(* Logix 5000 AddOnInstructionDefinition export Process_TU3VFDControl_Instance102_103; software revision 24.02 *)

TYPE FI_Data_IN :
STRUCT
   ConnectionFaulted : BOOL;
   RunMode : BOOL;
   Data : INT[6];   // Actual Values
END_STRUCT
END_TYPE

TYPE FI_Data_OUT :
STRUCT
   Data : INT[6];   // Control Data
END_STRUCT
END_TYPE

ADD_ON_INSTRUCTION Process_TU3VFDControl_Instance102_103   (* revision 1.1, vendor NORD Drivesystems, ExecutePrescan *)
// Control block for Nord VFD TU3 Instances 102/103
// Allows for control of up to eight (8) SK 5xxE VFDs.
// Revision note:
// Rev 1.1
// Better Ready Start Condition Logic
// Added Inhibited Output
// Added Fault Active Output
// Rev 1.0
VAR_IN_OUT
   FI_Status : _0342:TU3_EIP_DE5BFA94:I:0; {required}   // Input Data Map of VFD
   FI_Control : _0342:TU3_EIP_E8E6FFA2:O:0; {required}   // Output Data Map of VFD
END_VAR
VAR_INPUT
   Max_VFD_Number : SINT := 8;   // Maximum Number of VFDs on this specific node (1-8 for Instance 102/103)
   VFD_Number : SINT := 1; {visible}   // Number of VFD to control (1...Max_VFD_Number) for Instance 102/103)
   EnableFwd : BOOL; {visible}   // HIGH = Enable CW
   EnableRev : BOOL; {visible}   // HIGH = Enable CCW
   DisableVoltage : BOOL := 1; {visible}   // LOW = Output Voltage Disabled
   QuickStop : BOOL := 1; {visible}   // LOW = Emergency Stop Active
   FaultAckn : BOOL; {visible}   // Error / Fault Acknowledgement on Rising Edge
   ParameterSet : SINT; {visible}   // Parameter Set 1-4, If less than 1 or higher than 4, Set 1 as active
   Activate32BitSetpoint : BOOL; {visible}   // HIGH = Activate 32Bit Setpoint combining Setpoint 2 and 3
   ControlWordBit8_P480_11 : BOOL; {visible}   // Control Word Bit 8 Function set in P480[11]
   ControlWordBit9_P480_12 : BOOL; {visible}   // Control Word Bit 9 Function set in P480[12]
END_VAR
VAR_OUTPUT
   ControlWord : ALIAS FOR Control_Word; {access Read Only, visible}   // Control Word Read Only Version
END_VAR
VAR_INPUT
   Setpoint1 : INT; {visible}   // Setpoint 1 Function set in P546
   Setpoint2 : INT; {visible}   // Setpoint 2 Function set in P547, deactivated if "PositioningActiveBit" is set
   Setpoint3 : INT; {visible}   // Setpoint 3 Function set in P548, deactivated if "PositioningActiveBitt" is set
   Setpoint4 : INT;   // Setpoint 4 only available in SK 54xE
   Setpoint5 : INT;   // Setpoint 5 only available in SK 54xE
   Setpoint2_3_32 : DINT; {visible}   // 32 Bit Setpoint 2 & 3 combined for positioning
END_VAR
VAR_OUTPUT
   StatusWord : INT; {access Read Only, visible}   // Status Word
        .0   // Ready to Start
        .1   // Ready for Operation
        .2   // Operation Enabled
        .3   // Fault
        .4   // Voltage Enabled
        .5   // No Emergency Stop
        .6   // Starting Disabled
        .7   // Warning Active
        .8   // Setpoint Reached
        .9   // Bus Controller Active
        .10   // Function P481[9]
        .11   // Rotation Right Active
        .12   // Rotation Left Active
        .13   // Function P481[10]
        .14   // Parameter Set Bit 0
        .15   // Parameter Set Bit 1
   ActiveParameterSet : SINT; {access None, visible}   // Displays Active Parameter set
   CommunicationOK : BOOL; {access Read Only, visible}   // HIGH = Communication is OK
   ReadyToStart : BOOL; {access None, visible}   // HIGH = Drive Ready to Start
   VFD_Enabled : BOOL; {access None, visible}   // HIGH = VFD is Enabled
   Inhibited : BOOL; {access Read Only, visible}   // VFD is Inhibited
   Warning : BOOL; {access None, visible}   // HIGH = Drive has a warning
   Faulted : BOOL; {access None, visible}   // HIGH = Drive Faulted
   FaultActive : BOOL; {access Read Only, visible}   // Fault Conditions are Currently Active
   StatusWordBit10_P481_9 : BOOL; {access None, visible}   // Status Word Bit 10 Function set in P481[9]
   StatusWordBit13_P481_10 : BOOL; {access None, visible}   // Status Word Bit 13 Function set in P481[10]
   ActualValue1 : INT; {access None, visible}   // Actual Value 1 Function set in P543
   ActualValue2 : INT; {access None, visible}   // Actual Value 2 Function set in P544
   ActualValue3 : INT; {access None, visible}   // Actual Value 3 Function set in P545
   ActualValue4 : INT; {access None}   // Actual Value 4 only available in SK 54xE
   ActualValue5 : INT; {access None}   // Actual Value 5 only available in SK 54xE
   ActualValue2_3_32 : DINT; {access None, visible}   // 32 Bit Actual Value 2 & 3 Combined for Positioning
END_VAR
VAR
   Index : INT; {access None}   // Index of process data based on VFD_Number
   Control_Word : INT; {access Read Only}   // Control Word
        .0   // Enable Operation
        .1   // Disable Voltage (Low level disables voltage and stops VFD)
        .2   // Emergency Stop (Low level activates ESTOP and stops VFD)
        .3   // Ready for Operation
        .4   // Enable Pulses
        .5   // Enable Ramp
        .6   // Enable Setpoint
        .7   // Error Acknowledge
        .8   // Function P480[11]
        .9   // Function P480[12]
        .10   // Control Data Valid
        .11   // Rotation Direction Right
        .12   // Rotation Direction Left
        .13   // Reserved
        .14   // Parameter Set Bit 0
        .15   // Parameter Set Bit 1
   Control : FI_Data_OUT; {access None}
   Status : FI_Data_IN; {access None}
   LowWordOf32BitSetpoint : DINT; {access None}
   Temporary_Variable_32BitSepoint : DINT; {access None}
   HighWordOf32BitSetpoint : DINT; {access None}
   FI_Status_Size : INT; {access None}   // Size of Input Process Data
   FI_Control_Size : INT; {access None}   // Size of Output Process Data
END_VAR

ROUTINE Logic   (* ladder *)
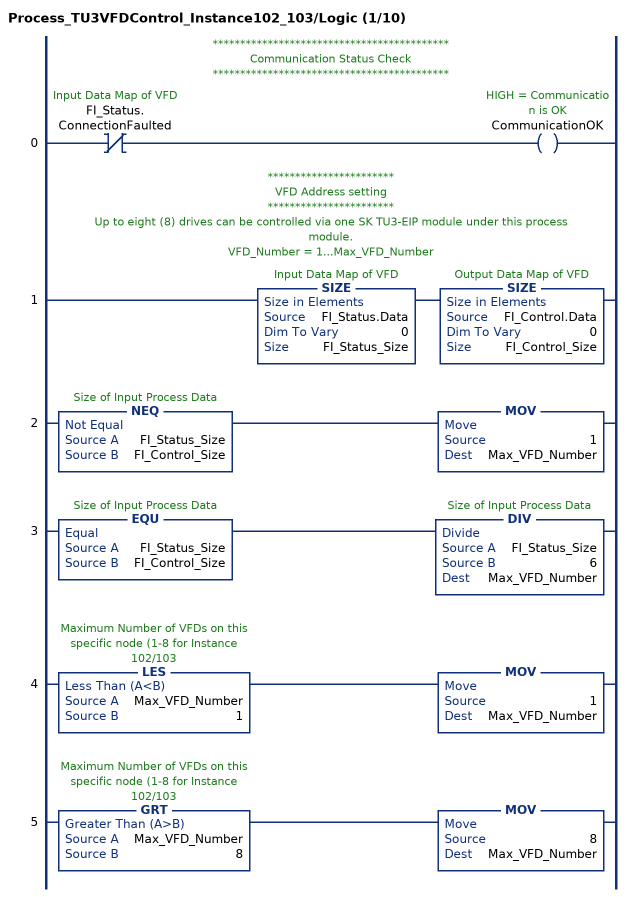
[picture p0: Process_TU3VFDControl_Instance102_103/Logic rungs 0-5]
   // *******************************************
   // Communication Status Check
   // *******************************************
   0: XIO(FI_Status.ConnectionFaulted)OTE(CommunicationOK);
   // ***********************
   // VFD Address setting
   // ***********************
   // Up to eight (8) drives can be controlled via one SK TU3-EIP module under this process module.
   // VFD_Number = 1...Max_VFD_Number
   1: SIZE(FI_Status.Data,0,FI_Status_Size)SIZE(FI_Control.Data,0,FI_Control_Size);
   2: NEQ(FI_Status_Size,FI_Control_Size)MOV(1,Max_VFD_Number);
   3: EQU(FI_Status_Size,FI_Control_Size)DIV(FI_Status_Size,6,Max_VFD_Number);
   4: LES(Max_VFD_Number,1)MOV(1,Max_VFD_Number);
   5: GRT(Max_VFD_Number,8)MOV(8,Max_VFD_Number);
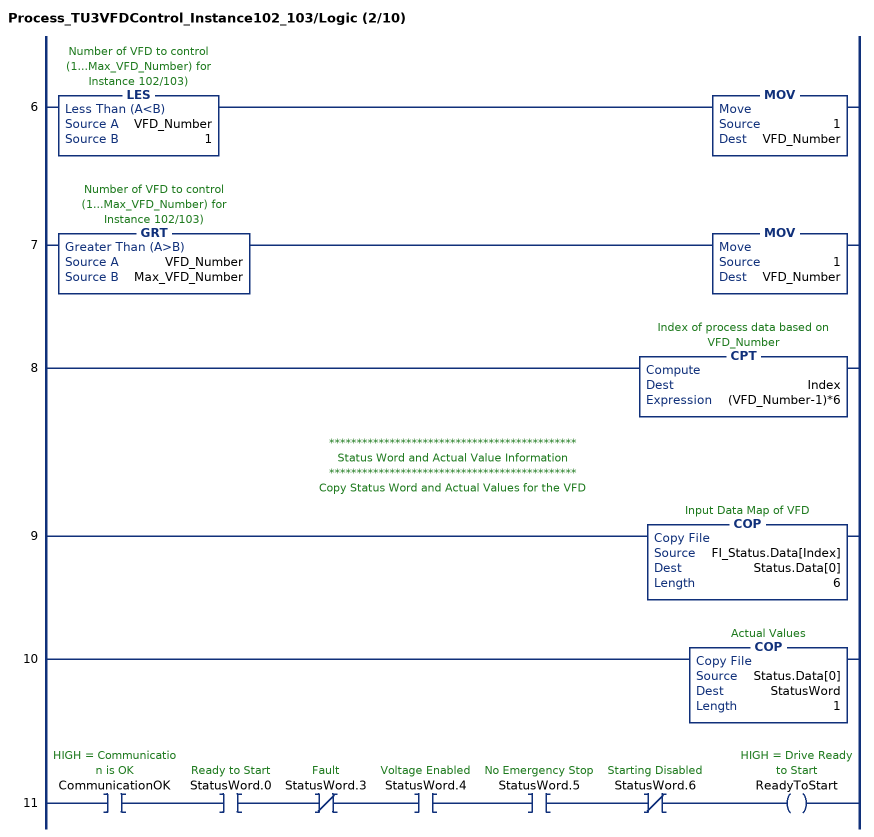
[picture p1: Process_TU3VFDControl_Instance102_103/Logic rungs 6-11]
   6: LES(VFD_Number,1)MOV(1,VFD_Number);
   7: GRT(VFD_Number,Max_VFD_Number)MOV(1,VFD_Number);
   8: CPT(Index,(VFD_Number-1)*6);
   // *********************************************
   // Status Word and Actual Value Information
   // *********************************************
   // Copy Status Word and Actual Values for the VFD
   9: COP(FI_Status.Data[Index],Status.Data[0],6);
   10: COP(Status.Data[0],StatusWord,1);
   11: XIC(CommunicationOK)XIC(StatusWord.0)XIO(StatusWord.3)XIC(StatusWord.4)XIC(StatusWord.5)XIO(StatusWord.6)OTE(ReadyToStart);
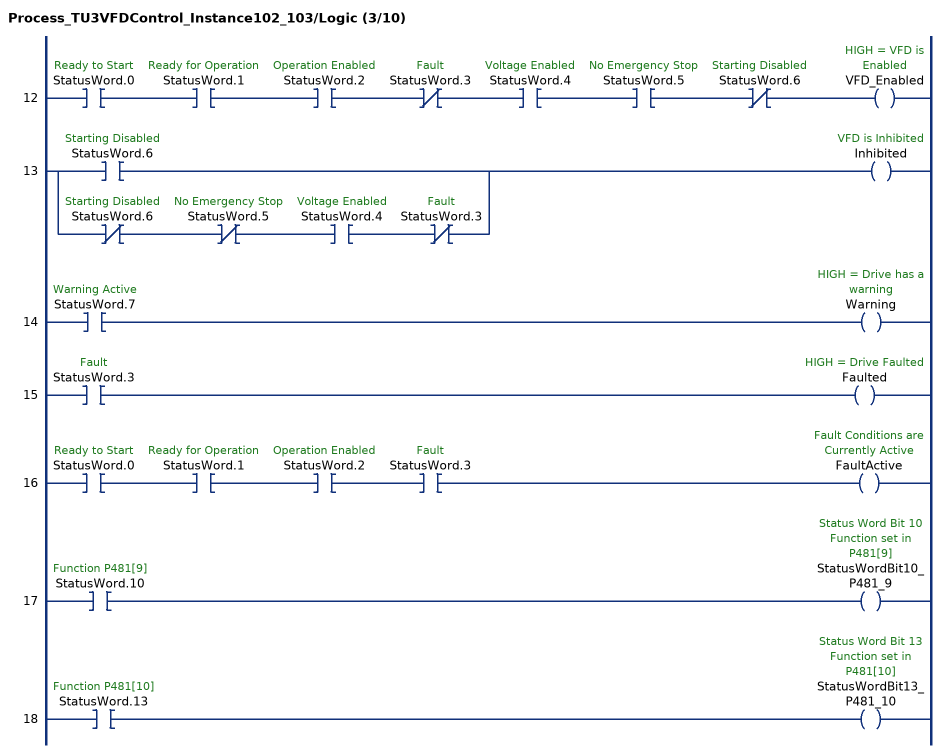
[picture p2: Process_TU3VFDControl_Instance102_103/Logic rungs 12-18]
   12: XIC(StatusWord.0)XIC(StatusWord.1)XIC(StatusWord.2)XIO(StatusWord.3)XIC(StatusWord.4)XIC(StatusWord.5)XIO(StatusWord.6)OTE(VFD_Enabled);
   13: [XIC(StatusWord.6) ,XIO(StatusWord.6) XIO(StatusWord.5) XIC(StatusWord.4) XIO(StatusWord.3) ]OTE(Inhibited);
   14: XIC(StatusWord.7)OTE(Warning);
   15: XIC(StatusWord.3)OTE(Faulted);
   16: XIC(StatusWord.0)XIC(StatusWord.1)XIC(StatusWord.2)XIC(StatusWord.3)OTE(FaultActive);
   17: XIC(StatusWord.10)OTE(StatusWordBit10_P481_9);
   18: XIC(StatusWord.13)OTE(StatusWordBit13_P481_10);
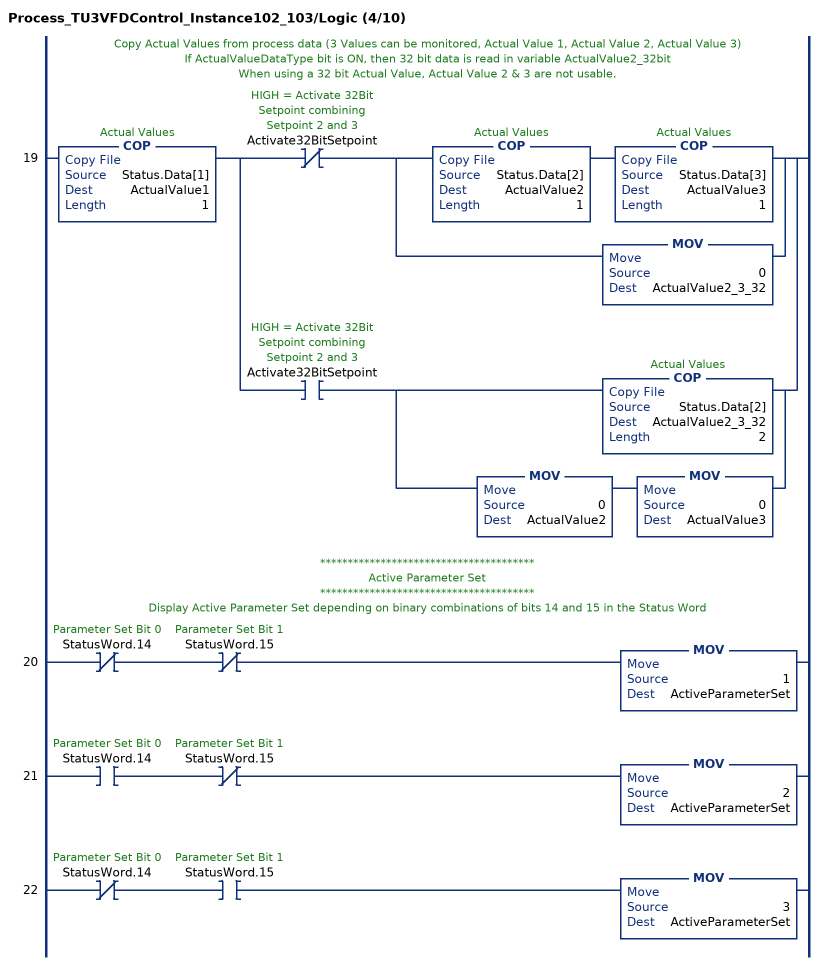
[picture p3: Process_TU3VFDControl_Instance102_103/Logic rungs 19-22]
   // Copy Actual Values from process data (3 Values can be monitored, Actual Value 1, Actual Value 2, Actual Value 3)
   // If ActualValueDataType bit is ON, then 32 bit data is read in variable ActualValue2_32bit
   // When using a 32 bit Actual Value, Actual Value 2 & 3 are not usable.
   19: COP(Status.Data[1],ActualValue1,1)[XIO(Activate32BitSetpoint) [COP(Status.Data[2],ActualValue2,1) COP(Status.Data[3],ActualValue3,1) ,MOV(0,ActualValue2_3_32) ] ,XIC(Activate32BitSetpoint) [COP(Status.Data[2],ActualValue2_3_32,2) ,MOV(0,ActualValue2) MOV(0,ActualValue3) ] ];
   // ***************************************
   // Active Parameter Set
   // ***************************************
   // Display Active Parameter Set depending on binary combinations of bits 14 and 15 in the Status Word
   20: XIO(StatusWord.14)XIO(StatusWord.15)MOV(1,ActiveParameterSet);
   21: XIC(StatusWord.14)XIO(StatusWord.15)MOV(2,ActiveParameterSet);
   22: XIO(StatusWord.14)XIC(StatusWord.15)MOV(3,ActiveParameterSet);
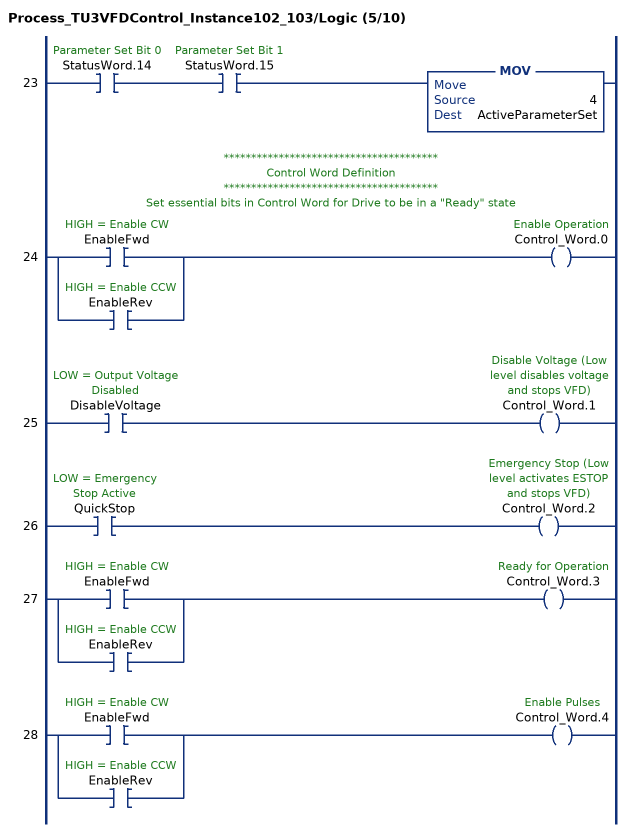
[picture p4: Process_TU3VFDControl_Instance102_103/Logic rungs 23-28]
   23: XIC(StatusWord.14)XIC(StatusWord.15)MOV(4,ActiveParameterSet);
   // ***************************************
   // Control Word Definition
   // ***************************************
   // Set essential bits in Control Word for Drive to be in a "Ready" state
   24: [XIC(EnableFwd) ,XIC(EnableRev) ]OTE(Control_Word.0);
   25: XIC(DisableVoltage)OTE(Control_Word.1);
   26: XIC(QuickStop)OTE(Control_Word.2);
   27: [XIC(EnableFwd) ,XIC(EnableRev) ]OTE(Control_Word.3);
   28: [XIC(EnableFwd) ,XIC(EnableRev) ]OTE(Control_Word.4);
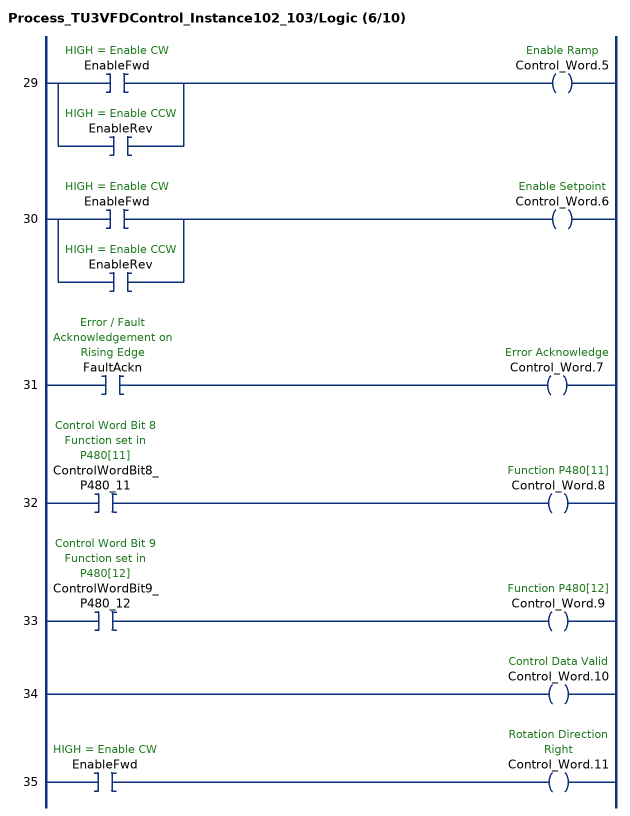
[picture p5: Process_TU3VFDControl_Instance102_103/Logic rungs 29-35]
   29: [XIC(EnableFwd) ,XIC(EnableRev) ]OTE(Control_Word.5);
   30: [XIC(EnableFwd) ,XIC(EnableRev) ]OTE(Control_Word.6);
   31: XIC(FaultAckn)OTE(Control_Word.7);
   32: XIC(ControlWordBit8_P480_11)OTE(Control_Word.8);
   33: XIC(ControlWordBit9_P480_12)OTE(Control_Word.9);
   34: OTE(Control_Word.10);
   35: XIC(EnableFwd)OTE(Control_Word.11);
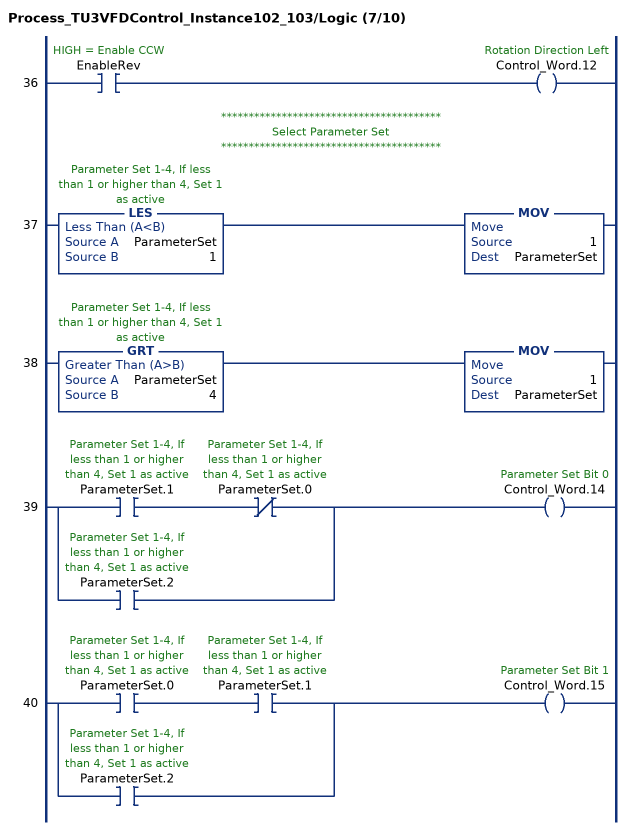
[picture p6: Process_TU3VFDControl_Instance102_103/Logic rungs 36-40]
   36: XIC(EnableRev)OTE(Control_Word.12);
   // ****************************************
   // Select Parameter Set
   // ****************************************
   37: LES(ParameterSet,1)MOV(1,ParameterSet);
   38: GRT(ParameterSet,4)MOV(1,ParameterSet);
   39: [XIC(ParameterSet.1) XIO(ParameterSet.0) ,XIC(ParameterSet.2) ]OTE(Control_Word.14);
   40: [XIC(ParameterSet.0) XIC(ParameterSet.1) ,XIC(ParameterSet.2) ]OTE(Control_Word.15);
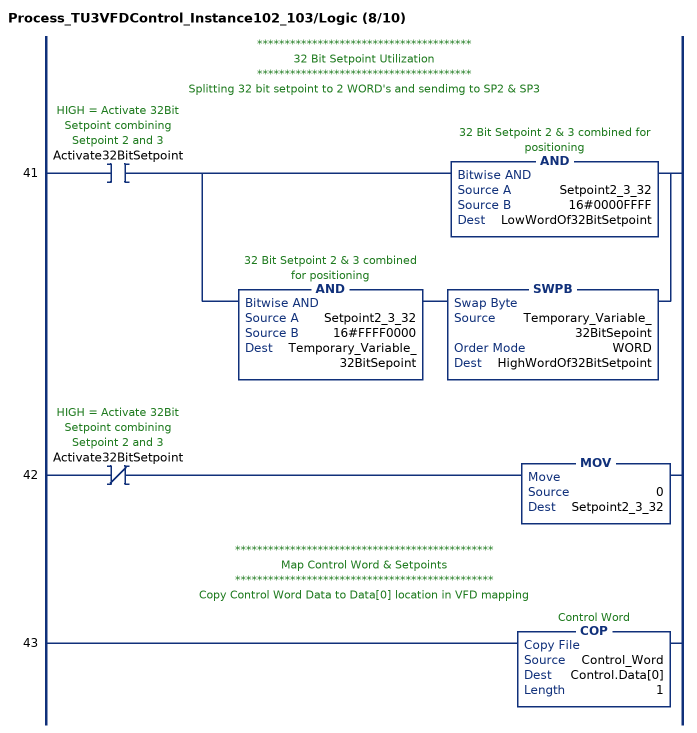
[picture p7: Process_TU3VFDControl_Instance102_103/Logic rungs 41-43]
   // ***************************************
   // 32 Bit Setpoint Utilization
   // ***************************************
   // Splitting 32 bit setpoint to 2 WORD's and sendimg to SP2 & SP3
   41: XIC(Activate32BitSetpoint)[AND(Setpoint2_3_32,16#0000FFFF,LowWordOf32BitSetpoint) ,AND(Setpoint2_3_32,16#FFFF0000,Temporary_Variable_32BitSepoint) SWPB(Temporary_Variable_32BitSepoint,WORD,HighWordOf32BitSetpoint) ];
   42: XIO(Activate32BitSetpoint)MOV(0,Setpoint2_3_32);
   // ***********************************************
   // Map Control Word & Setpoints
   // ***********************************************
   // Copy Control Word Data to Data[0] location in VFD mapping
   43: COP(Control_Word,Control.Data[0],1);
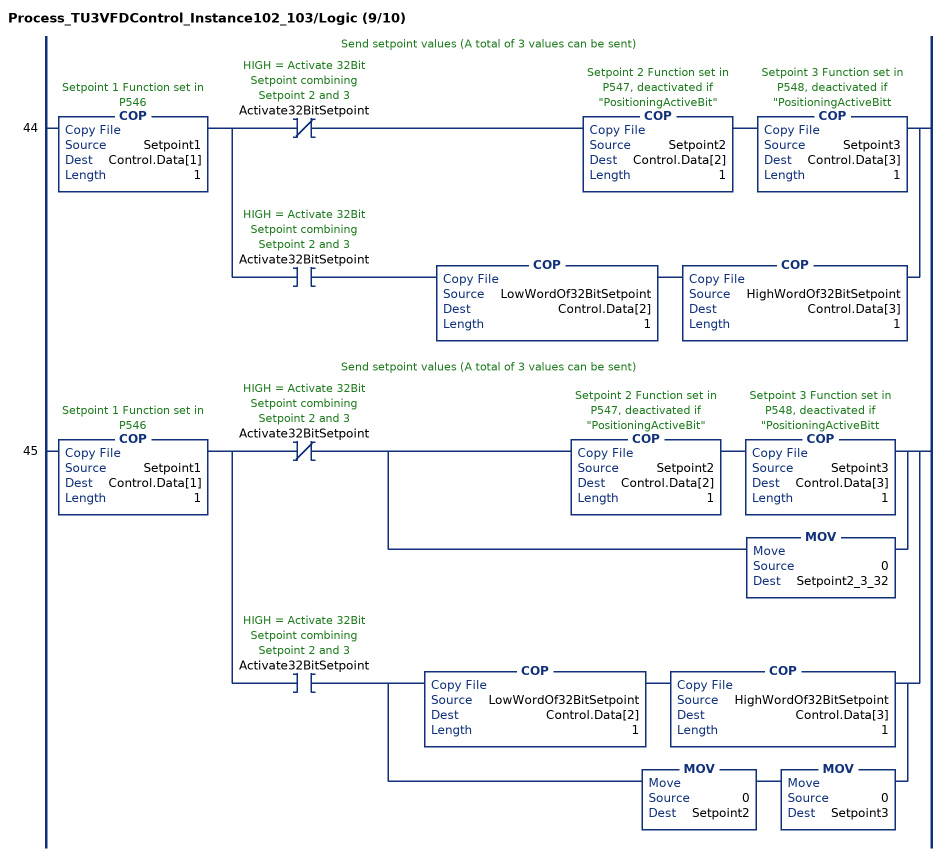
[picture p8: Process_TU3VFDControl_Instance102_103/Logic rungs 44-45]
   // Send setpoint values (A total of 3 values can be sent)
   44: COP(Setpoint1,Control.Data[1],1)[XIO(Activate32BitSetpoint) COP(Setpoint2,Control.Data[2],1) COP(Setpoint3,Control.Data[3],1) ,XIC(Activate32BitSetpoint) COP(LowWordOf32BitSetpoint,Control.Data[2],1) COP(HighWordOf32BitSetpoint,Control.Data[3],1) ];
   // Send setpoint values (A total of 3 values can be sent)
   45: COP(Setpoint1,Control.Data[1],1)[XIO(Activate32BitSetpoint) [COP(Setpoint2,Control.Data[2],1) COP(Setpoint3,Control.Data[3],1) ,MOV(0,Setpoint2_3_32) ] ,XIC(Activate32BitSetpoint) [COP(LowWordOf32BitSetpoint,Control.Data[2],1) COP(HighWordOf32BitSetpoint,Control.Data[3],1) ,MOV(0,Setpoint2) MOV(0,Setpoint3) ] ];
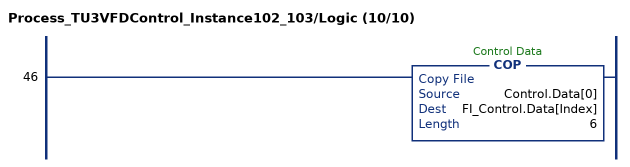
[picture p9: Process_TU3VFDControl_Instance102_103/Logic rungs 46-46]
   46: COP(Control.Data[0],FI_Control.Data[Index],6);
END_ROUTINE

ROUTINE Prescan   (* ladder *)
// Executed prior to first scan of AOI
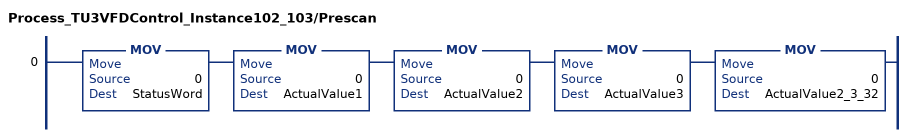
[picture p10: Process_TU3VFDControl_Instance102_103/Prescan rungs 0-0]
   0: MOV(0,StatusWord)MOV(0,ActualValue1)MOV(0,ActualValue2)MOV(0,ActualValue3)MOV(0,ActualValue2_3_32);
END_ROUTINE
END_ADD_ON_INSTRUCTION
